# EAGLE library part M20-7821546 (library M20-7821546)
M20: 15 Pos Receptacle SIL Straight 3mm THT Connector 8.5mm high Tin Source: Datasheet
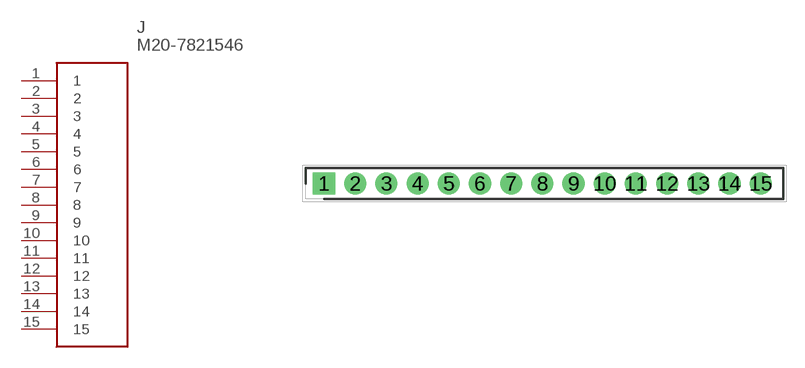
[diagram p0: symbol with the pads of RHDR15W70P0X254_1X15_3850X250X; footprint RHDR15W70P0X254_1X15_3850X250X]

Designator prefix J

## M20-7821546 (Description: M20: 15 Pos Receptacle SIL Straight 3mm THT Connector 8.5mm high Tin; Height: 8.5mm; Manufacturer_Name: Harwin; Manufacturer_Part_Number: M20-7821546; Mouser_Part_Number: 855-M20-7821546; Mouser_Price-Stock: https://www.mouser.co.uk/ProductDetail/Harwin/M20-7821546?qs=ulE8k0yEMYaXNbedAzK8cQ%3D%3D)  [RHDR15W70P0X254_1X15_3850X250X]
1  1
2  2
3  3
4  4
5  5
6  6
7  7
8  8
9  9
10  10
11  11
12  12
13  13
14  14
15  15

## Footprint RHDR15W70P0X254_1X15_3850X250X (pad centres in mm)
M20-7821546
drill 1.2 pad 1.8 square: 1 0,0
drill 1.2 pad 1.8: 2 2.54,0; 3 5.08,0; 4 7.62,0; 5 10.16,0; 6 12.7,0; 7 15.24,0; 8 17.78,0; 9 20.32,0; 10 22.86,0; 11 25.4,0; 12 27.94,0; 13 30.48,0; 14 33.02,0; 15 35.56,0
